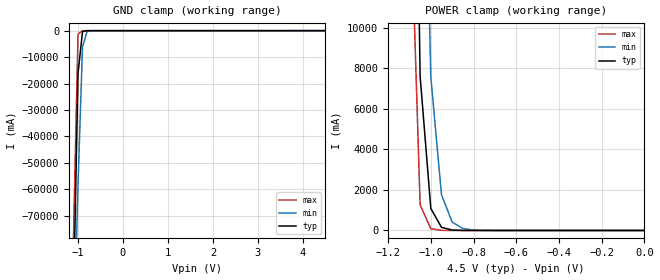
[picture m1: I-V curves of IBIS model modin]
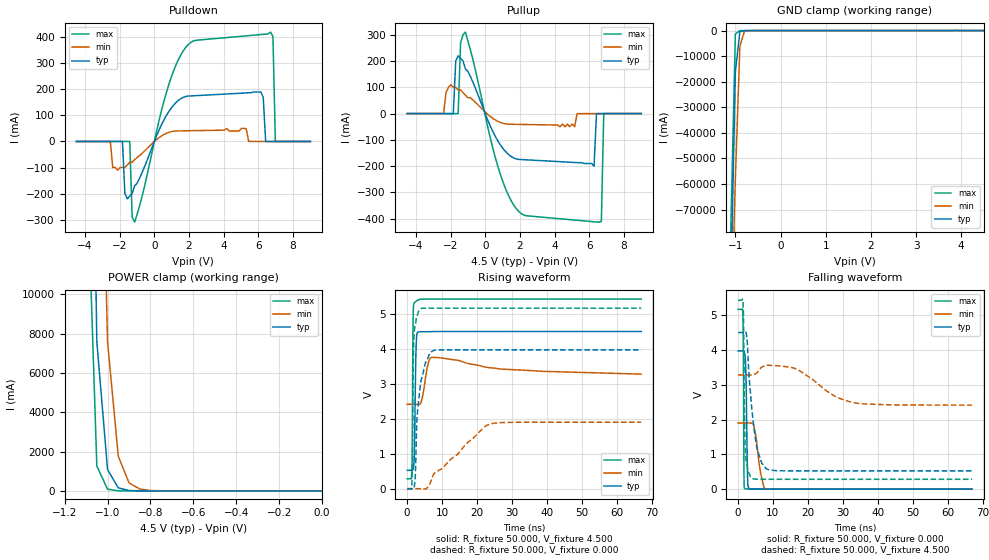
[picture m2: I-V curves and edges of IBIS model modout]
| IBIS file 54ac574.ibs created by s2ibis3 verion 1.1
| North Carolina State University, ERL, 2006
[IBIS ver] 4.0
[File name] 54ac574_4v5_die_rev1.ibs
[File Rev] 1.0
[Date]  12 Jun 2009
[Source] CAD & Design Solution (Catania) - STMicroelectronics
[Notes]
  (Note1) This IBIS model is the model of product in dice form(it doesn't
   include any component from package and bounding);
  (Note2) This IBIS model is extracted with nominal 4.5V power supply
   (min:3.0V, typ:4.5V, max:5.5V);
  (Note3) This model has few Warnings about the non-monotonicity
   of I-V curves, but they are not indicative of problems
   inside the model;
[Copyright] (c) 2009 STMicroelectronics
|   Component 54AC574
[Component] 54AC574
[Manufacturer] STMicroelectronics
[Package]
| variable  typ   min   max
R_pkg   0.0   0.0   0.0
L_pkg   0.0H   0.0H   0.0H
C_pkg   0.0F   0.0F   0.0F
[Pin]  signal_name   model_name   R_pin   L_pin   C_pin
OEN   OEN   modin   0.0   0.0   0.0
D0   D0   modin   0.0   0.0   0.0
D1   D1   modin   0.0   0.0   0.0
D2   D2   modin   0.0   0.0   0.0
D3   D3   modin   0.0   0.0   0.0
D4   D4   modin   0.0   0.0   0.0
D5   D5   modin   0.0   0.0   0.0
D6   D6   modin   0.0   0.0   0.0
D7   D7   modin   0.0   0.0   0.0
GND   GND   GND   0.0   0.0   0.0
CP   CP   modin   0.0   0.0   0.0
O7   O7   modout   0.0   0.0   0.0
O6   O6   modout   0.0   0.0   0.0
O5   O5   modout   0.0   0.0   0.0
O4   O4   modout   0.0   0.0   0.0
O3   O3   modout   0.0   0.0   0.0
O2   O2   modout   0.0   0.0   0.0
O1   O1   modout   0.0   0.0   0.0
O0   O0   modout   0.0   0.0   0.0
VCC   VCC   POWER   0.0   0.0   0.0
| Models and submodels in the file (2): modin (Input), modout (3-state)
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|   Model modin
[Model]  modin
Model_type Input
Vinl =   1.3500V
Vinh =   3.1500V
C_comp   0.5317pF   NA   NA
[Temperature Range]   25.0000   0.1250k   -55.0000
[Voltage Range]   4.5000V   3.0000V   5.5000V
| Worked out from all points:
|   GND clamp passes 1 mA (typ) near -0.71 V on its own axis
|   POWER clamp passes 1 mA (typ) near -0.81 V on its own axis
[GND_clamp]
|Voltage   I(typ)   I(min)   I(max)
-4.5V     -3.016kA   -2.305kA   -4.061kA
-1.1V     -101.1A    -122.4A    -77.32A
-1V       -16.28A    -58.17A    -1.327A
-900mV    -332.5mA   -6.163A    -6.557mA
-800mV    -6.845mA   -334.5mA   -32.39uA
-700mV    -140.8uA   -18.25mA   -158nA
4.5V      9.691nA    319.5nA    7pA
[POWER_clamp]
|Voltage   I(typ)   I(min)   I(max)
-4.5V     2.956kA    2.246kA    4.002kA
-1.1V     41.46A     62.72A     18.07A
-1.05V    7.601A     30.62A     1.265A
-1V       1.086A     7.577A     88.65mA
-950mV    155.3mA    1.765A     6.25mA
-900mV    22.27mA    411.2mA    440.6uA
-850mV    3.204mA    95.92mA    30.86uA
-800mV    459.7uA    22.42mA    2.159uA
0V        4.5pA      41.65pA    5.5pA
|   Model modout
[Model]  modout
Model_type 3-state
Polarity   Non-Inverting
Enable   Active-Low
Vmeas = 2.25V
Cref = 50pF
Rref = 500
C_comp   2.7906pF   NA   NA
[Temperature Range]   25.0000   0.1250k   -55.0000
[Voltage Range]   4.5000V   3.0000V   5.5000V
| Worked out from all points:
|   slope of the pulldown table from 0 to 0.675 V, typ, clamps not added: 6.92 ohm
|   slope of the pullup table from 0 to 0.675 V, typ, clamps not added: 6.92 ohm
|   GND clamp passes 1 mA (typ) near -0.71 V on its own axis
|   POWER clamp passes 1 mA (typ) near -0.81 V on its own axis
|   rising waveform, R_fixture 50.000, V_fixture 4.500: 20-80 % time 362ps typ, 882ps min, 191ps max; typ from 0.527 V to 4.5 V
|   rising waveform, R_fixture 50.000, V_fixture 0.000: 20-80 % time 1.75ns typ, 12.3ns min, 316ps max; typ from 0 V to 3.97 V
|   falling waveform, R_fixture 50.000, V_fixture 0.000: 20-80 % time 356ps typ, 1.54ns min, 143ps max; typ from 3.97 V to 0 V
|   falling waveform, R_fixture 50.000, V_fixture 4.500: 20-80 % time 2.28ns typ, 7.76ns min, 387ps max; typ from 4.5 V to 0.527 V
[Pulldown]
|Voltage   I(typ)   I(min)   I(max)
-4.5V     0A         0A         0A
-1.84V    0A         -100mA     0A
-1.7V     -200mA     -100mA     0A
-1.42V    -210mA     -80mA      0A
-1.28V    -200mA     -80mA      -290mA
-1.14V    -170mA     -70mA      -310mA
1.8V      172.6mA    41mA       360.5mA
6.14V     190mA      0A         410.6mA
6.7V      0A         0A         420mA
6.84V     0A         0A         403.1mA
6.98V     0A         0A         0A
9V        0A         0A         0A
[Pullup]
|Voltage   I(typ)   I(min)   I(max)
-4.5V     0A         0A         0A
-1.84V    0A         100mA      0A
-1.56V    220mA      90mA       0A
-1.42V    210mA      90mA       270mA
-1.14V    170mA      70mA       310mA
1.66V     -169.2mA   -40.7mA    -349.3mA
6.28V     -200mA     0A         -411.5mA
6.42V     0A         0A         -412.3mA
6.56V     0A         0A         -413mA
6.7V      0A         0A         -410mA
6.84V     0A         0A         0A
9V        0A         0A         0A
[GND_clamp]
|Voltage   I(typ)   I(min)   I(max)
-4.5V     -3.016kA   -2.305kA   -4.061kA
-1.1V     -101.1A    -122.4A    -77.32A
-1V       -16.28A    -58.17A    -1.327A
-900mV    -332.1mA   -6.162A    -6.494mA
-800mV    -6.775mA   -334.1mA   -31.78uA
-700mV    -138.2uA   -18.12mA   -155.6nA
4.5V      4.5pA      319.5uA    3.5pA
[POWER_clamp]
|Voltage   I(typ)   I(min)   I(max)
-4.5V     2.956kA    2.246kA    4.002kA
-1.1V     41.46A     62.72A     18.07A
-1.05V    7.6A       30.62A     1.264A
-1V       1.085A     7.577A     88.45mA
-950mV    155mA      1.764A     6.188mA
-900mV    22.14mA    410.8mA    432.9uA
-850mV    3.162mA    95.66mA    30.29uA
-800mV    451.7uA    22.27mA    2.119uA
0V        4.5pA      41.65pA    5.5pA
[Ramp]
| variable   typ   min   max
dV/dt_r  2.3850/0.3647n   0.8052/1.2897n   3.0866/0.1887n
dV/dt_f  2.3835/0.3555n   1.1414/1.5570n   3.0993/0.1418n
R_load = 50.0000
[Rising Waveform]
R_fixture = 50.000
V_fixture = 4.500
|  time   V(typ)   V(min)   V(max)
0s        526.6mV    2.416V     283.7mV
1.35ns    525.9mV    2.416V     529.3mV
1.425ns   526.1mV    2.416V     943.8mV
1.65ns    547.7mV    2.416V     4.488V
1.875ns   648.8mV    2.416V     5.281V
2.1ns     1.306V     2.417V     5.328V
2.475ns   3.764V     2.416V     5.354V
2.7ns     4.353V     2.414V     5.379V
6.9ns     4.496V     3.756V     5.428V
67ns      4.5V       3.28V      5.427V
[Rising Waveform]
R_fixture = 50.000
V_fixture = 0.000
|  time   V(typ)   V(min)   V(max)
0s        466.9uV    641.9uV    380.8uV
1.275ns   936.4uV    641.8uV    33.88mV
1.5ns     -2.716mV   638.1uV    616.3mV
1.725ns   -10.99mV   631.7uV    3.602V
1.875ns   -2.157mV   627.4uV    4.206V
2.85ns    2.092V     854.7uV    4.962V
3.75ns    2.945V     -565.6uV   5.149V
7.2ns     3.938V     327mV      5.167V
23.77ns   3.973V     1.851V     5.167V
67ns      3.973V     1.903V     5.166V
[Falling Waveform]
R_fixture = 50.000
V_fixture = 0.000
|  time   V(typ)   V(min)   V(max)
0s        3.973V     1.903V     5.166V
1.35ns    3.973V     1.903V     5.098V
1.5ns     3.975V     1.903V     4.458V
1.725ns   3.97V      1.903V     154.5mV
2.025ns   3.832V     1.903V     10.09mV
2.325ns   3.022V     1.903V     5.684mV
2.775ns   216.9mV    1.903V     5.652mV
3.3ns     7.876mV    1.906V     5.115mV
7.5ns     2.088mV    24.73mV    458.6uV
67ns      466.9uV    641.9uV    380.8uV
[Falling Waveform]
R_fixture = 50.000
V_fixture = 4.500
|  time   V(typ)   V(min)   V(max)
0s        4.5V       3.281V     5.428V
1.425ns   4.499V     3.281V     5.392V
1.575ns   4.503V     3.281V     4.999V
1.8ns     4.519V     3.281V     2.475V
2.025ns   4.536V     3.281V     1.284V
3.9ns     2.371V     3.282V     320.1mV
5.475ns   1.153V     3.351V     285.4mV
8.925ns   555.5mV    3.56V      283.7mV
33.15ns   526.6mV    2.485V     283.7mV
67ns      526.8mV    2.416V     283.7mV
